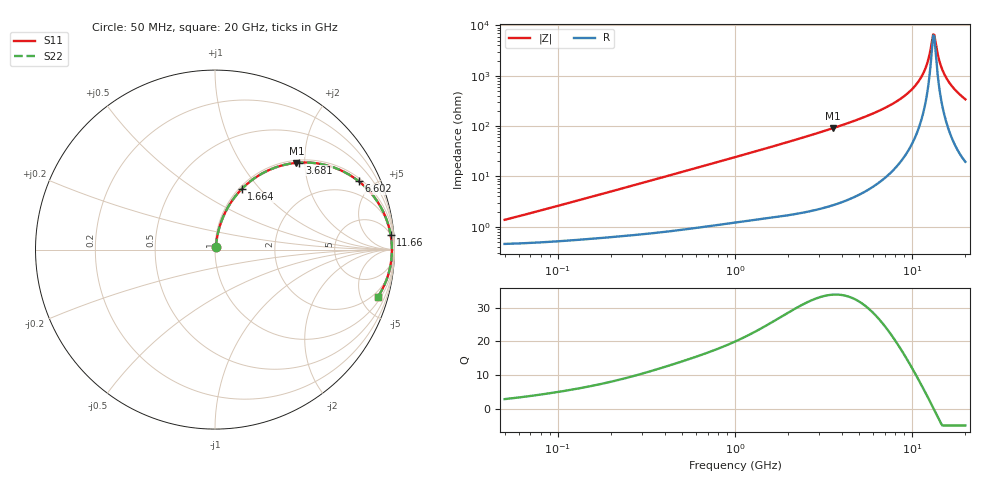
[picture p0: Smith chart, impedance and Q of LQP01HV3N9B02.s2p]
!Murata Part Number: LQP01HV3N9B02
!These Parameters are Measured in Series Mode Connection
!  o--[Z]--o
!Port1  Port2
!  o-------o
!Freq. Start=50[MHz] Stop=20[GHz], 401[Steps]
# Hz S RI R 50
!Freq.(Hz) S11(Real) S11(Imag) S21(Real) S21(Imag) S12(Real) S12(Imag) S22(Real) S22(Imag)
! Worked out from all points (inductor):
!   401 points, 50 MHz to 20 GHz, reference 50 ohm
!   read as one part in series: L = 4.11 nH near 53.89 MHz
!   highest Q = 33.9 at 3.572 GHz (marker M1), where L = 4.05 nH
!   self-resonance near 13.15 GHz
!   S11 on the Smith chart (normalised r, x): 50 MHz: 1.01, +0.03; 1.664 GHz: 1.03, +0.80; 3.681 GHz: 1.06, +1.88; 6.602 GHz: 1.16, +4.12; 11.66 GHz: 5, +23; 20 GHz: 1.39, -6.79
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5e7  0.00471 0.0128  0.9953 -0.0128  0.9953 -0.0128  0.00471 0.0128
1.364002e8  0.00672 0.0341  0.9933 -0.0341  0.9933 -0.0341  0.00672 0.0341
3.721004e8  0.0158 0.0894  0.9842 -0.0894  0.9842 -0.0894  0.0158 0.0894
1e9  0.0651 0.2228  0.9349 -0.2228  0.9349 -0.2228  0.0651 0.2228
1.664083e9  0.1484 0.3369  0.8516 -0.3369  0.8516 -0.3369  0.1484 0.3369
2.728004e9  0.3172 0.4502  0.6828 -0.4502  0.6828 -0.4502  0.3172 0.4502
3.572216e9  0.4536 0.4833  0.5464 -0.4833  0.5464 -0.4833  0.4536 0.4833
3.680849e9  0.4703 0.4846  0.5297 -0.4846  0.5297 -0.4846  0.4703 0.4846
4.966507e9  0.6447 0.4632  0.3553 -0.4632  0.3553 -0.4632  0.6447 0.4632
6.601595e9  0.8006 0.381  0.1994 -0.381  0.1994 -0.381  0.8006 0.381
7.442007e9  0.856 0.3298  0.144 -0.3298  0.144 -0.3298  0.856 0.3298
9.892087e9  0.9511 0.1793  0.0489 -0.1793  0.0489 -0.1793  0.9511 0.1793
1.082228e10  0.969 0.1257  0.031 -0.1257  0.031 -0.1257  0.969 0.1257
1.166392e10  0.979 0.0797  0.021 -0.0797  0.021 -0.0797  0.979 0.0797
1.220001e10  0.9829 0.0516  0.0171 -0.0516  0.0171 -0.0516  0.9829 0.0516
1.295331e10  0.9855 0.0138  0.0145 -0.0138  0.0145 -0.0138  0.9855 0.0138
1.334722e10  0.9857 -0.00522  0.0143 0.00522  0.0143 0.00522  0.9857 -0.00522
1.354865e10  0.9855 -0.0148  0.0145 0.0148  0.0145 0.0148  0.9855 -0.0148
1.438523e10  0.9829 -0.053  0.0171 0.053  0.0171 0.053  0.9829 -0.053
1.550395e10  0.9752 -0.101  0.0248 0.101  0.0248 0.101  0.9752 -0.101
1.747767e10  0.9522 -0.1773  0.0478 0.1773  0.0478 0.1773  0.9522 -0.1773
2e10  0.9077 -0.2622  0.0923 0.2622  0.0923 0.2622  0.9077 -0.2622
